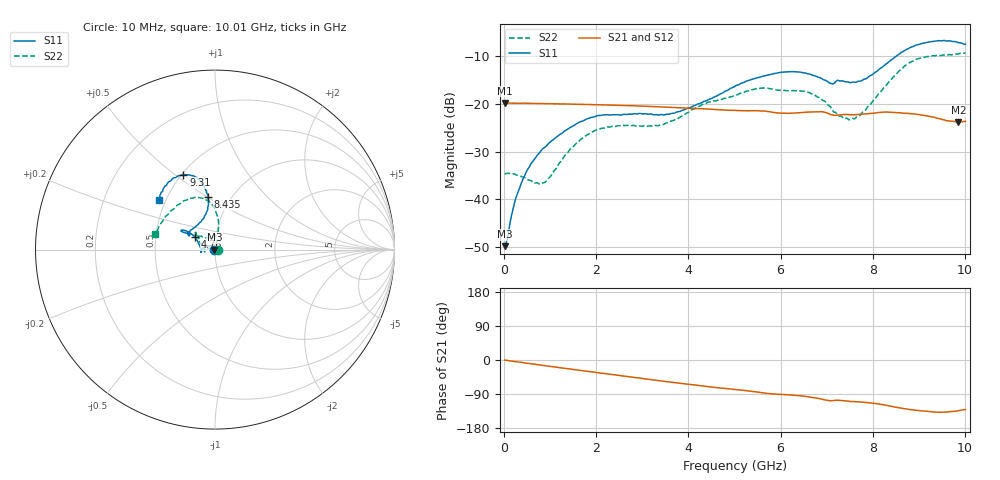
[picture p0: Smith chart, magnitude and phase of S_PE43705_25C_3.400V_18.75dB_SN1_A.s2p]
! Device ID: PE43705
! Serial: 1
! Insertion: A
! Impedance: 50 ohm
! Temp: 25C
! VDD: 3.400V
! Attenuation Step: 18.75dB
#  Hz  S  RI  R  50
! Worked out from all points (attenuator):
!   401 points, 10 MHz to 10.01 GHz, reference 50 ohm
!   highest |S21| = -19.82 dB at 10 MHz (marker M1); lowest = -23.8 dB at 9.86 GHz (marker M2)
!   lowest |S11| = -49.8 dB at 10 MHz (marker M3), VSWR 1.01, Z = 49.7 + j0.0408 ohm
!   |S11| at or under -10 dB: start of sweep to 8.513 GHz
!   |S22| runs from -36.9 to -9.3 dB; largest |S21 - S12| = 0.0013
!   S11 on the Smith chart (normalised r, x): 10 MHz: 0.99, +0.00; 4.76 GHz: 0.79, +0.11; 8.435 GHz: 0.78, +0.50; 9.31 GHz: 0.51, +0.54; 10.01 GHz: 0.46, +0.31
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1e7  -0.0032 0.000411  0.1021 -0.000426  0.1022 -0.000348  0.0184 0.000244
2.6e8  -0.00468 0.0094  0.1012 -0.00799  0.1011 -0.00797  0.0166 0.00695
5.6e8  -0.0128 0.0183  0.0996 -0.0168  0.0996 -0.0168  0.00884 0.013
9.1e8  -0.0288 0.0214  0.0969 -0.0267  0.0969 -0.0265  -0.00661 0.0139
1.685e9  -0.065 0.0078  0.0871 -0.0463  0.0871 -0.0463  -0.0432 0.000611
2.21e9  -0.0763 -0.00841  0.0782 -0.0578  0.0782 -0.0577  -0.0557 -0.0104
3.36e9  -0.0761 -0.00681  0.0537 -0.0758  0.0539 -0.0757  -0.0593 0.0029
3.86e9  -0.0833 0.0176  0.0425 -0.0801  0.0424 -0.08  -0.0707 0.0232
4.76e9  -0.1115 0.0701  0.0229 -0.083  0.0229 -0.0831  -0.0924 0.0659
5.01e9  -0.1274 0.0851  0.018 -0.0833  0.0181 -0.0835  -0.0984 0.0742
5.535e9  -0.159 0.1024  0.00701 -0.084  0.00715 -0.084  -0.1119 0.0919
5.985e9  -0.1831 0.1089  -0.000811 -0.0798  -0.000615 -0.0797  -0.1053 0.0899
6.685e9  -0.1755 0.0957  -0.0127 -0.0813  -0.0127 -0.0813  -0.099 0.0782
7.11e9  -0.1409 0.0809  -0.0227 -0.0734  -0.0225 -0.0733  -0.0556 0.0686
7.535e9  -0.1067 0.1291  -0.0255 -0.0726  -0.0251 -0.0727  -0.0115 0.0691
7.785e9  -0.0738 0.1621  -0.0285 -0.0726  -0.0283 -0.0725  0.00528 0.082
8.36e9  -0.0359 0.2763  -0.0423 -0.07  -0.0421 -0.0699  0.0162 0.1719
8.435e9  -0.0387 0.2939  -0.0443 -0.0681  -0.0443 -0.0684  0.0128 0.1876
8.86e9  -0.0893 0.3873  -0.0519 -0.0591  -0.0511 -0.0592  -0.0473 0.2751
9.31e9  -0.1761 0.4168  -0.0532 -0.0495  -0.0531 -0.0493  -0.1499 0.2816
9.86e9  -0.2909 0.3252  -0.0444 -0.0464  -0.0446 -0.0461  -0.297 0.1517
1.001e10  -0.3147 0.2791  -0.0427 -0.0497  -0.0431 -0.05  -0.3321 0.0878
